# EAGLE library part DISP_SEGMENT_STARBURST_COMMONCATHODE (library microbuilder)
Starburst Segment Display - Common Cathode 0.8" Red Alphanumeric LED Display - BL-S80A-13UHR-11
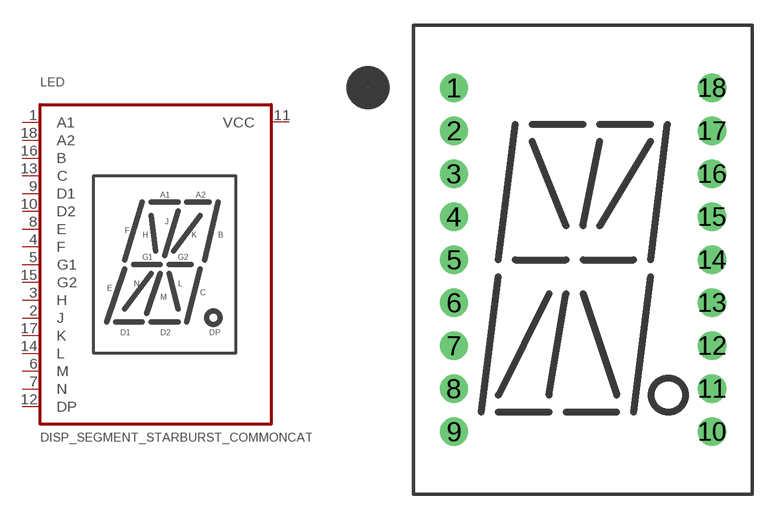
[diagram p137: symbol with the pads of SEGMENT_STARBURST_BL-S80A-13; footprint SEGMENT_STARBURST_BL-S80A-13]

Designator prefix LED

## DISP_SEGMENT_STARBURST_COMMONCATHODEBLS80A13  [SEGMENT_STARBURST_BL-S80A-13]
1  A1
2  J
3  H
4  F
5  G1
6  M
7  N
8  E
9  D1
10  D2
11  VCC  pwr
12  DP
13  C
14  L
15  G2
16  B
17  K
18  A2

## Footprint SEGMENT_STARBURST_BL-S80A-13 (pad centres in mm)
drill 0.8 pad 1.676: 1 -7.62,10.16; 2 -7.62,7.62; 3 -7.62,5.08; 4 -7.62,2.54; 5 -7.62,0; 6 -7.62,-2.54; 7 -7.62,-5.08; 8 -7.62,-7.62; 9 -7.62,-10.16; 10 7.62,-10.16; 11 7.62,-7.62; 12 7.62,-5.08; 13 7.62,-2.54; 14 7.62,0; 15 7.62,2.54; 16 7.62,5.08; 17 7.62,7.62; 18 7.62,10.16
